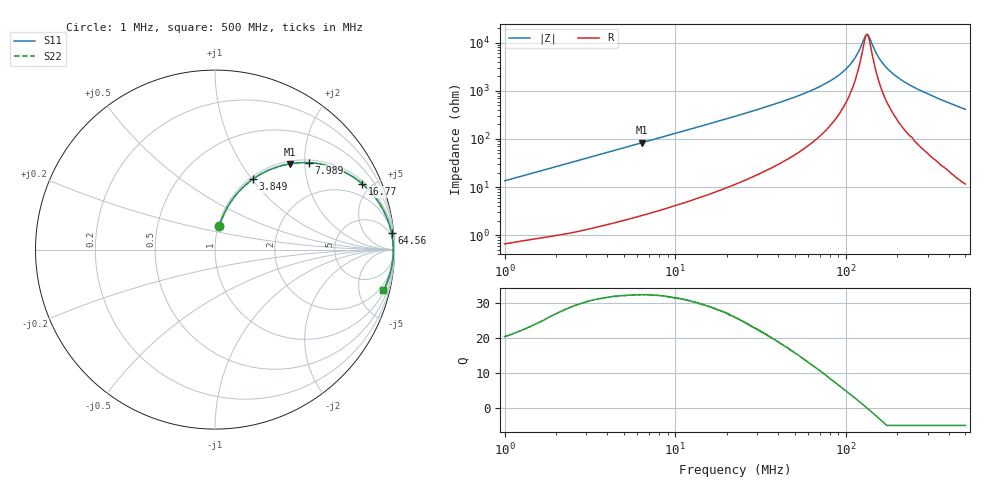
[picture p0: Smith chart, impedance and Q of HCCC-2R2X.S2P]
!s-Parameter Generated by FASTRON Sdn. Bhd.
!FASTRON P/N : HCCC-2R2X
!Keysight Technologies,E4991B,MY54100416,A.01.15
!Date: Thu Apr 02 14:12:09 2026
!Version  : Rev00 Thu Apr 02 14:12:09 2026
!Data & Calibration Information:
!PortZ  Port1:50+j0  Port2:50+j0
!When reading, reference impedance value at option line is always used.
!Remarks : This data is being provided solely for informational purposes.
!Freq	S11	S21	S12	S22
# Hz S dB R 50
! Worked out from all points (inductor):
!   1601 points, 1 MHz to 500 MHz, reference 50 ohm
!   read as one part in series: L = 2.13 uH near 1.032 MHz
!   highest Q = 32.5 at 6.402 MHz (marker M1), where L = 2.09 uH
!   self-resonance near 132.5 MHz
!   S11 on the Smith chart (normalised r, x): 1 MHz: 1.01, +0.27; 3.849 MHz: 1.03, +1.01; 7.989 MHz: 1.06, +2.09; 16.77 MHz: 1.15, +4.40; 64.56 MHz: 3, +21; 500 MHz: 1.23, -8.22
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1000000  -17.51 79.6  -0.13 -7.6  -0.13 -7.6  -17.51 79.6
2820919  -9.22 67.9  -0.66 -20.2  -0.66 -20.2  -9.22 67.9
3848922  -7.00 61.7  -1.10 -26.5  -1.10 -26.5  -7.00 61.7
6402024  -3.97 49.0  -2.44 -39.3  -2.44 -39.3  -3.97 49.0
7957584  -2.97 43.0  -3.32 -45.2  -3.32 -45.2  -2.97 43.0
7988553  -2.96 42.9  -3.34 -45.3  -3.34 -45.3  -2.96 42.9
1.677481e7  -0.93 24.1  -7.77 -63.9  -7.77 -63.9  -0.93 24.1
2.236068e7  -0.57 18.4  -9.99 -69.4  -9.99 -69.4  -0.57 18.4
4.05111e7  -0.21 9.9  -15.32 -77.1  -15.32 -77.1  -0.21 9.9
6.307767e7  -0.11 5.5  -20.37 -79.9  -20.37 -79.9  -0.11 5.5
6.456494e7  -0.10 5.3  -20.68 -79.9  -20.68 -79.9  -0.10 5.3
8.440921e7  -0.08 3.2  -25.07 -79.5  -25.07 -79.5  -0.08 3.2
1.013146e8  -0.07 1.9  -29.59 -76.0  -29.59 -76.0  -0.07 1.9
1.138355e8  -0.06 1.0  -34.20 -68.5  -34.20 -68.5  -0.06 1.0
1.284016e8  -0.06 0.2  -42.22 -30.2  -42.22 -30.2  -0.06 0.2
1.319406e8  -0.06 0.0  -43.45 -5.6  -43.45 -5.6  -0.06 0.0
1.371661e8  -0.06 -0.2  -42.20 30.7  -42.20 30.7  -0.06 -0.2
1.5714e8  -0.06 -1.2  -33.36 71.1  -33.36 71.1  -0.06 -1.2
1.77937e8  -0.06 -2.1  -28.73 77.7  -28.73 77.7  -0.06 -2.1
2.110998e8  -0.07 -3.4  -24.57 80.2  -24.57 80.2  -0.07 -3.4
2.583476e8  -0.09 -5.1  -21.05 80.7  -21.05 80.7  -0.09 -5.1
5e8  -0.31 -13.6  -12.59 74.8  -12.59 74.8  -0.31 -13.6
